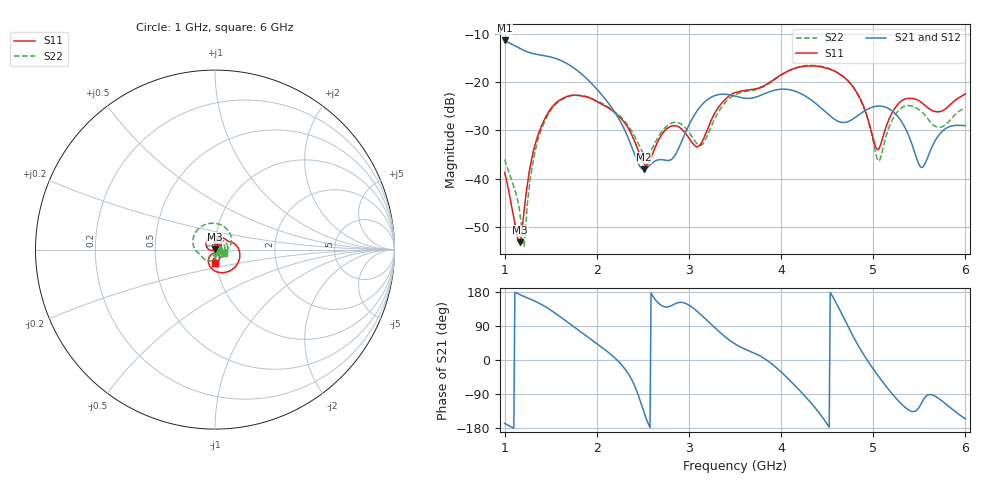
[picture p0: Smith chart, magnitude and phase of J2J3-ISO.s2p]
!Agilent Technologies,E8364B,MY43040528,A.07.50.67
!Agilent E8364B: A.07.50.67
!Date: Sunday, March 01, 2026 15:34:01
!Correction: S11(Full 2 Port(1,2))
!S21(Full 2 Port(1,2))
!S12(Full 2 Port(1,2))
!S22(Full 2 Port(1,2))
!S2P File: Measurements: S11, S21, S12, S22:
# Hz S  dB  R 50
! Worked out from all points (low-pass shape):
!   451 points, 1 GHz to 6 GHz, reference 50 ohm
!   highest |S21| = -11.30 dB at 1 GHz (marker M1); lowest = -38.1 dB at 2.511 GHz (marker M2)
!   |S21| within 3 dB of the highest: start of sweep to 1.383 GHz
!   lowest |S11| = -53.3 dB at 1.167 GHz (marker M3), VSWR 1.00, Z = 49.9 + j0.159 ohm
!   |S11| at or under -10 dB: start of sweep to end of sweep
!   |S22| runs from -54.1 to -16.5 dB; largest |S21 - S12| = 0.00098
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1e9  -38.75 35.5  -11.30 -167.4  -11.33 -167.3  -36.06 -16.8
1.166667e9  -53.29 132.6  -12.98 172.4  -13.01 172.4  -47.27 6.4
1.211111e9  -46.72 -176.8  -13.39 167.6  -13.42 167.7  -54.06 75.2
1.3e9  -35.34 -164.5  -13.99 158.4  -14.02 158.5  -37.42 129.0
1.411111e9  -28.57 176.4  -14.38 145.0  -14.41 145.0  -29.24 105.9
1.577778e9  -23.97 139.9  -15.20 118.7  -15.23 118.7  -24.18 61.9
1.844444e9  -22.85 88.5  -18.42 70.9  -18.45 71.0  -22.78 -1.7
2.266667e9  -27.59 33.8  -28.52 -12.1  -28.54 -12.2  -27.30 -74.2
2.511111e9  -36.89 41.9  -38.10 -137.3  -38.14 -137.2  -34.86 -79.1
2.666667e9  -32.15 82.6  -36.12 150.7  -36.15 150.7  -31.41 -55.2
2.866667e9  -29.08 58.0  -34.58 150.2  -34.61 150.3  -28.31 -89.4
3.133333e9  -32.67 80.9  -24.83 118.9  -24.87 118.9  -33.10 -95.5
3.5e9  -22.16 56.5  -22.86 42.4  -22.90 42.5  -22.60 -122.4
4.044444e9  -17.96 6.4  -21.43 -41.7  -21.46 -41.7  -18.00 165.6
4.344444e9  -16.58 -40.2  -23.92 -118.8  -23.96 -118.8  -16.49 107.8
4.788889e9  -21.17 -113.1  -27.51 59.2  -27.55 59.2  -21.14 14.3
5.055556e9  -33.97 -86.7  -24.93 -42.5  -24.97 -42.5  -36.35 21.4
5.166667e9  -27.86 -54.3  -25.45 -77.7  -25.48 -77.6  -29.55 58.7
5.322222e9  -23.66 -72.6  -28.63 -120.0  -28.67 -119.9  -25.11 30.5
5.522222e9  -24.17 -97.4  -37.70 -114.5  -37.74 -114.5  -26.04 -9.2
5.722222e9  -26.10 -90.5  -30.72 -103.5  -30.75 -103.5  -29.34 -11.0
6e9  -22.42 -91.0  -29.01 -155.1  -29.05 -155.1  -25.21 -22.5
